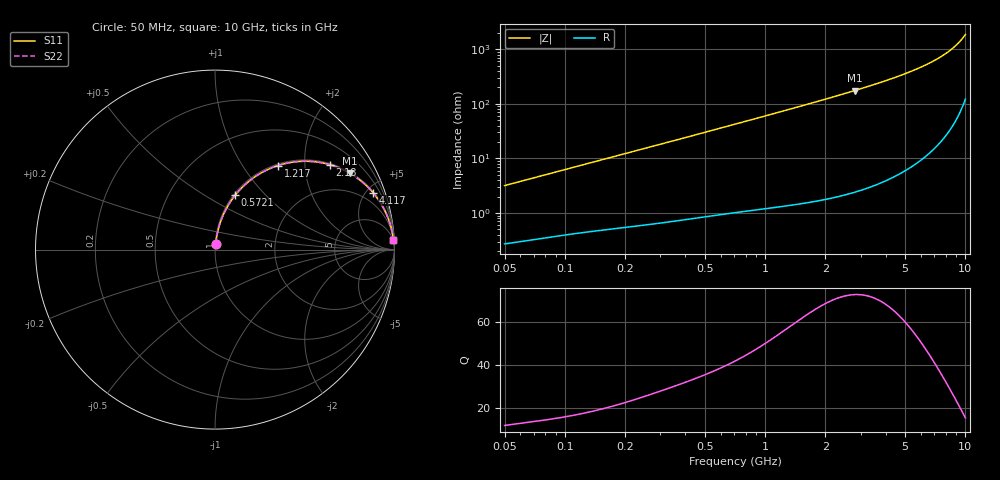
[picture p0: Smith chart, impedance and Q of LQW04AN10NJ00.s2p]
!Murata Part Number: LQW04AN10NJ00
!These Parameters are Measured in Series Mode Connection
!  o--[Z]--o
!Port1  Port2
!  o-------o
!Freq. Start=50[MHz] Stop=10[GHz], 401[Steps]
# Hz S RI R 50
!Freq.(Hz)	S 11(Real)	S 11(Imag)	S 21(Real)	S 21(Imag)	S 12(Real)	S 12(Imag)	S 22(Real)	S 22(Imag)
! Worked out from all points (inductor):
!   401 points, 50 MHz to 10 GHz, reference 50 ohm
!   read as one part in series: L = 10 nH near 51.34 MHz
!   highest Q = 72.9 at 2.804 GHz (marker M1), where L = 9.97 nH
!   S11 on the Smith chart (normalised r, x): 50 MHz: 1.01, +0.06; 572.1 MHz: 1.02, +0.69; 1.217 GHz: 1.03, +1.46; 2.18 GHz: 1.04, +2.67; 4.117 GHz: 1.08, +5.52; 10 GHz: 3, +37
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5e7  0.0037 0.0315  0.9963 -0.0315  0.9963 -0.0315  0.0037 0.0315
1.214486e8  0.00986 0.0739  0.9901 -0.0739  0.9901 -0.0739  0.00986 0.0739
1.930779e8  0.0188 0.115  0.9812 -0.115  0.9812 -0.115  0.0188 0.115
2.949953e8  0.0368 0.171  0.9632 -0.171  0.9632 -0.171  0.0368 0.171
4.218272e8  0.0671 0.2354  0.9329 -0.2354  0.9329 -0.2354  0.0671 0.2354
5.720629e8  0.1121 0.3025  0.8879 -0.3025  0.8879 -0.3025  0.1121 0.3025
7.071068e8  0.1585 0.3534  0.8415 -0.3534  0.8415 -0.3534  0.1585 0.3534
9.215873e8  0.2387 0.416  0.7613 -0.416  0.7613 -0.416  0.2387 0.416
1.21714e9  0.3512 0.4684  0.6488 -0.4684  0.6488 -0.4684  0.3512 0.4684
1.717543e9  0.5197 0.492  0.4803 -0.492  0.4803 -0.492  0.5197 0.492
2.179987e9  0.6392 0.4732  0.3608 -0.4732  0.3608 -0.4732  0.6392 0.4732
2.803837e9  0.7522 0.4249  0.2478 -0.4249  0.2478 -0.4249  0.7522 0.4249
3.420121e9  0.8257 0.3725  0.1743 -0.3725  0.1743 -0.3725  0.8257 0.3725
4.116968e9  0.8802 0.3174  0.1198 -0.3174  0.1198 -0.3174  0.8802 0.3174
4.171863e9  0.8836 0.3133  0.1164 -0.3133  0.1164 -0.3133  0.8836 0.3133
5.657692e9  0.9448 0.2193  0.0552 -0.2193  0.0552 -0.2193  0.9448 0.2193
6.458996e9  0.9626 0.1791  0.0374 -0.1791  0.0374 -0.1791  0.9626 0.1791
7.181012e9  0.9738 0.1476  0.0262 -0.1476  0.0262 -0.1476  0.9738 0.1476
7.878683e9  0.9815 0.1206  0.0185 -0.1206  0.0185 -0.1206  0.9815 0.1206
8.530394e9  0.9867 0.0977  0.0133 -0.0977  0.0133 -0.0977  0.9867 0.0977
9.114482e9  0.9901 0.0789  0.00985 -0.0789  0.00985 -0.0789  0.9901 0.0789
1e10  0.9937 0.0528  0.00629 -0.0528  0.00629 -0.0528  0.9937 0.0528
